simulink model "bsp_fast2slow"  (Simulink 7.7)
settings: Solver=FixedStepDiscrete  StartTime=0.0  StopTime=20.0  RelTol=1e-3

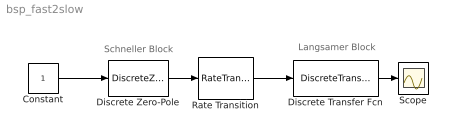
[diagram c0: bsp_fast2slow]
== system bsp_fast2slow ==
  note: Langsamer Block
  note: Schneller Block
  Constant : Constant
  Discrete Transfer Fcn : DiscreteTransferFcn  Denominator=[1 0.5 1]  SampleTime=2
  Discrete Zero-Pole : DiscreteZeroPole  Poles=[0 0 0.1]  Gain=2
  Rate Transition : RateTransition
  Scope : Scope
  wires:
  Discrete Transfer Fcn/1 -> Scope/1
  Constant/1 -> Discrete Zero-Pole/1
  Discrete Zero-Pole/1 -> Rate Transition/1
  Rate Transition/1 -> Discrete Transfer Fcn/1
